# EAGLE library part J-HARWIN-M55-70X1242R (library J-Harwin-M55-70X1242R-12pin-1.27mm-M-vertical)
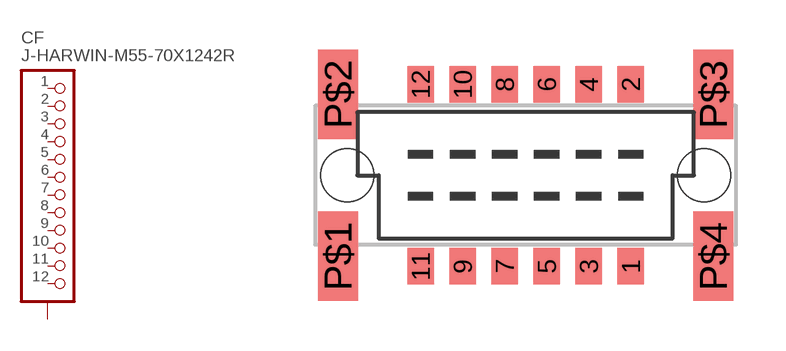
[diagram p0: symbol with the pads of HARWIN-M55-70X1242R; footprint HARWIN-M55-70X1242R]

Designator prefix CF

## J-HARWIN-M55-70X1242R  [HARWIN-M55-70X1242R]
1  1  pas
2  2  pas
3  3  pas
4  4  pas
5  5  pas
6  6  pas
7  7  pas
8  8  pas
9  9  pas
10  10  pas
11  11  pas
12  12  pas
P$1  SHIELDS  pas
P$2  SHIELDS  pas
P$3  SHIELDS  pas
P$4  SHIELDS  pas

## Footprint HARWIN-M55-70X1242R (pad centres in mm)
smd 0.8 x 1.1: 1 3.175,-2.75; 2 3.175,2.75; 3 1.905,-2.75; 4 1.905,2.75; 5 0.635,-2.75; 6 0.635,2.75; 7 -0.635,-2.75; 8 -0.635,2.75; 9 -1.905,-2.75; 10 -1.905,2.75; 11 -3.175,-2.75; 12 -3.175,2.75
smd 1.2 x 2.7: P$1 -5.67,-2.45; P$2 -5.67,2.45; P$3 5.67,2.45; P$4 5.67,-2.45
hole 1.6 at -5.385,0
hole 1.6 at 5.385,0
